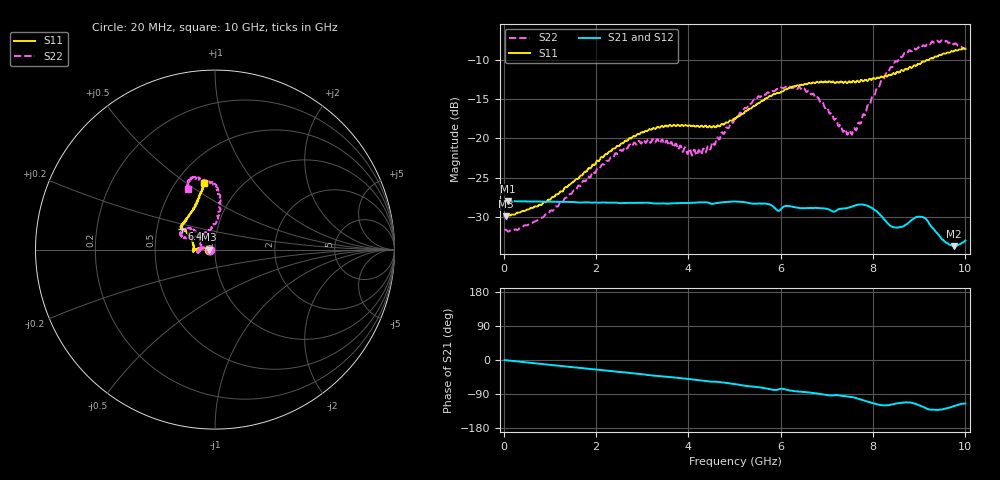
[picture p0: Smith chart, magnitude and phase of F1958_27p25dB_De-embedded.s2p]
! Integrated Device Technology
! Corporate Headquarters
! 6024 Silver Creek Valley Road
! San Jose, CA 95138  USA
! Phone:  1-408-284-8200
! Toll Free:  1-800-223-1366
! Webpage:  http://www.idt.com/
! Timing and RF Division
! 515 Groton Road, Suite 102
! Westford, MA 01886-6024
! Device:  F1958
! Description: 7-bit 0.25 dB Digital Step Attenuator
! Frequency:  0.001 -  6.000 GHz
! Package:  4x4 mm Thin QFN Plastic Package: 24 pin
! Ports:  2 RF, 12 DC
!  Pin  1  = D0
!  Pin  2  = VDD
!  Pin  3  = VMODE
!  Pin  4  = GND
!  Pin  5  = RF1  =  Port 1
!  Pin  6  = GND
!  Pin  7  = GND
!  Pin  8  = GND
!  Pin  9  = GND
!  Pin 10  = GND
!  Pin 11  = GND
!  Pin 12  = GND
!  Pin 13  = GND
!  Pin 14  = RF2  =  Port 2
!  Pin 15  = GND
!  Pin 16  = LE
!  Pin 17  = CLK
!  Pin 18  = DATA
!  Pin 19  = D6
!  Pin 20  = D5
!  Pin 21  = D4
!  Pin 22  = D3
!  Pin 23  = D2
!  Pin 24  = D1
! State:  109
! Atten State:  27.25 dB
! Voltage:  +3.30 Volts
! Current:  0.258 mA
! Data:  The device was measured on a F1958 evaluation board which has
!  individual transmission lines to the RF pins.  Data was collected
!  using a calibrated network analyzer.  The evaluation board was
!  de-embedded using Automatic Fixture Removal (AFR).
!  The reference plane is the edge of the package pin.
! Misc:
!  Action Tracker AT0419
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# GHz S dB R 50
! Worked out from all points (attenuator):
!   500 points, 20 MHz to 10 GHz, reference 50 ohm
!   highest |S21| = -28.01 dB at 100 MHz (marker M1); lowest = -33.8 dB at 9.76 GHz (marker M2)
!   lowest |S11| = -30.0 dB at 40 MHz (marker M3), VSWR 1.07, Z = 46.9 - j0.0415 ohm
!   |S11| at or under -10 dB: start of sweep to 9.154 GHz
!   |S22| runs from -31.9 to -7.5 dB; largest |S21 - S12| = 0.00029
!   S11 on the Smith chart (normalised r, x): 20 MHz: 0.94, -0.00; 6.4 GHz: 0.67, +0.17; 10 GHz: 0.68, +0.58
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0.02  -29.92 -178.9  -28.04 -0.3  -28.03 -0.3  -31.69 -179.0
0.04  -29.95 -179.2  -28.02 -0.5  -28.03 -0.4  -31.66 -178.5
0.1  -29.84 179.2  -28.01 -1.3  -28.02 -1.2  -31.90 179.9
0.84  -28.35 170.8  -28.07 -10.7  -28.07 -10.7  -30.12 172.1
1.7  -24.72 170.6  -28.18 -21.3  -28.18 -21.2  -25.66 171.0
2.62  -20.36 176.6  -28.24 -32.7  -28.22 -32.8  -21.11 180.0
3.36  -18.62 -176.1  -28.31 -42.3  -28.32 -42.5  -20.43 -170.1
4.24  -18.55 -179.5  -28.18 -53.2  -28.19 -53.3  -21.53 168.1
4.5  -18.61 174.6  -28.35 -57.2  -28.37 -57.2  -20.87 150.7
5.02  -17.47 160.2  -28.06 -64.0  -28.07 -64.0  -17.32 137.7
5.58  -15.21 150.1  -28.33 -72.7  -28.34 -72.7  -14.60 139.5
5.94  -14.18 148.0  -29.24 -77.9  -29.26 -78.0  -13.69 148.3
6.4  -13.24 147.5  -28.90 -83.4  -28.91 -83.4  -13.41 155.4
6.68  -12.89 146.4  -28.89 -86.7  -28.90 -86.6  -14.35 157.4
7.5  -12.74 138.0  -28.80 -97.0  -28.80 -97.0  -18.98 119.2
7.68  -12.70 135.1  -28.46 -102.0  -28.46 -101.9  -18.01 99.0
7.9  -12.50 128.7  -28.66 -110.6  -28.64 -110.6  -15.70 88.8
8.34  -11.87 118.6  -30.97 -119.1  -30.98 -119.2  -11.48 83.5
8.66  -11.38 112.9  -31.24 -112.3  -31.22 -112.4  -9.26 87.4
9.08  -10.15 107.0  -30.05 -123.6  -30.07 -123.6  -8.10 98.6
9.76  -8.80 100.0  -33.77 -121.5  -33.80 -121.3  -7.92 111.3
10  -8.52 99.8  -33.04 -114.8  -33.06 -114.5  -8.63 113.7
